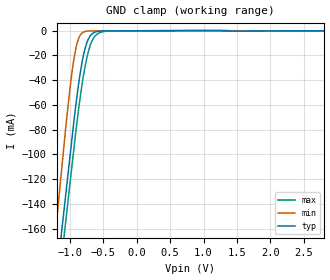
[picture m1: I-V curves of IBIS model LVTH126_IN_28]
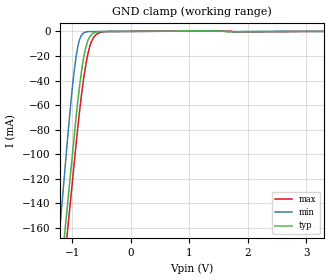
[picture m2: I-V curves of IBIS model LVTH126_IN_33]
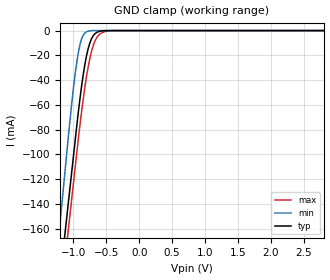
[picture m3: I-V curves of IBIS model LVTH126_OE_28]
| TEXAS INSTRUMENTS INCORPORATED
| Standard Linear and Logic Group
| IBIS Model of SN74LVTH126
| 3.3-V ABT QUADRUPLE BUS BUFFERS WITH 3-STATE OUTPUTS
| This file contains package information for the following:
|  TSSOP 14-pin (PW) package as [Component] LVTH126_PW
|  SOP 14-pin (NS) package as [Component] LVTH126_NS
|  TVSOP 14-pin (DGV) package as [Component] LVTH126_DGV
|  SSOP 14-pin (DB) package as [Component] LVTH126_DB
|  SOIC 14-pin (D) package as [Component] LVTH126_D
| This device can be powered at the following Vccs:
|  2.8 volt Vcc
|  3.3 volt Vcc
| This file provides unique models under the [Model Selector] for each Vcc.
| For operation at a specific Vcc, select the appropriate model after each
| [Model Selector] keyword.
[IBIS Ver]   3.2
[Comment char]  |_char
[File Name]   sn74lvth126.ibs
[File Rev]   1.1 | b_die
[Date]   June 13, 2002
[Source]   Data created from TI-SPICE simulations at TI-SLL.
[Notes]   The following is an IBIS list for the SN74LVTH126.
   Please contact sllibis@ti.com with questions and
   comments concerning SLL IBIS models.
   - Due to the fact that the device is 5-V input/output
   tolerant, the output model has some non-monotonic
   warnings.
   - C_comp values are taken at a different test condition
   than the Ci in data sheet.
   - Power clamp data has been deleted since there is no
   power clamp diode in the device.
   - Due to presence of BUS HOLD at input, GND-CLAMP curves
   have non-monotonic warnings.
[Disclaimer] Property of Texas Instruments Incorporated.  Unauthorized
   reproduction and/or distribution is strictly prohibited.
   This product is protected under copyright law.
   Created 2002, (C) Copyright 2002, Texas Instruments
   Incorporated, All Rights Reserved
   UNLESS THERE IS A SIGNED, WRITTEN AGREEMENT TO THE
   CONTRARY, TEXAS INSTRUMENTS (TI) IS PROVIDING THE IBIS
   MODELS  AND WITHOUT ANY WARRANTY, EXPRESSED OR
   IMPLIED. TI assumes no liability for:
   1) the accuracy of the IBIS models provided to your
   company;
   2) the proper functioning of these IBIS Models in your
   design or for any resulting applications; or
   3) infringement of patents, copyrights or intellectual
   property rights resulting from your use of these IBIS
   models.
   TI provides IBIS Models as a service to our customers.
   You and your company shall not distribute, sell or give
   these models to anyone else without prior written
   permission from TI.
   TI reserves the right to make changes to our products or
   to discontinue any semiconductor product or service
   without notice, and advises our customers to obtain the
   latest version of relevant information to verify, before
   placing orders, that the information being relied on is
   current.
   Please be aware that your receipt and use of the IBIS
   information provided shall serve as acceptance of these
   terms and conditions. If you do not accept these terms,
   you should return or destroy the IBIS models and any
   other accompanying information immediately.
| Component LVTH126_PW 14-pin TSSOP
[Component]   LVTH126_PW
[Manufacturer]  Texas Instruments, Inc.
[Package]
|   typ   min   max
R_pkg   3.200e-02   2.900e-02   3.500e-02
L_pkg   2.378e-09   2.170e-09   2.680e-09
C_pkg   3.140e-13   2.700e-13   3.350e-13
[Pin]   signal_name   model_name   R_pin   L_pin   C_pin
1   1OE   LVTH126_OE   3.300e-02   2.618e-09   3.300e-13
2   1A   LVTH126_IN   3.100e-02   2.313e-09   3.170e-13
3   1Y   LVTH126_OUT   3.000e-02   2.310e-09   3.140e-13
4   2OE   LVTH126_OE   3.100e-02   2.173e-09   2.720e-13
5   2A   LVTH126_IN   3.000e-02   2.204e-09   3.090e-13
6   2Y   LVTH126_OUT   3.200e-02   2.315e-09   3.170e-13
7   GND   GND   3.500e-02   2.680e-09   3.350e-13
8   3Y   LVTH126_OUT   3.300e-02   2.640e-09   3.330e-13
9   3A   LVTH126_IN   3.400e-02   2.347e-09   3.190e-13
10   3OE   LVTH126_OE   2.900e-02   2.277e-09   3.130e-13
11   4Y   LVTH126_OUT   3.100e-02   2.170e-09   2.700e-13
12   4A   LVTH126_IN   3.100e-02   2.244e-09   3.110e-13
13   4OE   LVTH126_OE   3.300e-02   2.343e-09   3.210e-13
14   VCC   POWER   3.500e-02   2.657e-09   3.320e-13
| Component LVTH126_NS 14-pin SOP
[Component]   LVTH126_NS
[Manufacturer]  Texas Instruments, Inc.
[Package]
|   typ   min   max
R_pkg   4.500e-02   3.900e-02   5.400e-02
L_pkg   3.796e-09   2.561e-09   4.952e-09
C_pkg   5.280e-13   2.880e-13   7.100e-13
[Pin]   signal_name   model_name   R_pin   L_pin   C_pin
1   1OE   LVTH126_OE   4.700e-02   4.867e-09   7.060e-13
2   1A   LVTH126_IN   5.100e-02   4.083e-09   5.920e-13
3   1Y   LVTH126_OUT   4.100e-02   2.915e-09   3.760e-13
4   2OE   LVTH126_OE   3.900e-02   2.561e-09   2.880e-13
5   2A   LVTH126_IN   4.100e-02   3.101e-09   4.300e-13
6   2Y   LVTH126_OUT   4.700e-02   4.047e-09   5.890e-13
7   GND   GND   5.100e-02   4.909e-09   7.000e-13
8   3Y   LVTH126_OUT   4.500e-02   4.784e-09   6.940e-13
9   3A   LVTH126_IN   5.400e-02   4.176e-09   5.970e-13
10   3OE   LVTH126_OE   3.900e-02   3.287e-09   4.490e-13
11   4Y   LVTH126_OUT   3.900e-02   2.586e-09   2.940e-13
12   4A   LVTH126_IN   4.000e-02   2.802e-09   3.710e-13
13   4OE   LVTH126_OE   4.900e-02   4.080e-09   5.930e-13
14   VCC   POWER   5.200e-02   4.952e-09   7.100e-13
| Component LVTH126_DGV 14-pin TVSOP
[Component]   LVTH126_DGV
[Manufacturer]  Texas Instruments, Inc.
[Package]
|   typ   min   max
R_pkg   3.500e-02   2.000e-02   4.500e-02
L_pkg   2.499e-09   2.077e-09   2.966e-09
C_pkg   3.610e-13   3.050e-13   4.160e-13
[Pin]   signal_name   model_name   R_pin   L_pin   C_pin
1   1OE   LVTH126_OE   2.700e-02   2.717e-09   3.730e-13
2   1A   LVTH126_IN   3.700e-02   2.434e-09   3.980e-13
3   1Y   LVTH126_OUT   3.400e-02   2.200e-09   3.160e-13
4   2OE   LVTH126_OE   2.000e-02   2.077e-09   3.090e-13
5   2A   LVTH126_IN   3.000e-02   2.147e-09   3.050e-13
6   2Y   LVTH126_OUT   4.200e-02   2.580e-09   4.080e-13
7   GND   GND   3.900e-02   2.921e-09   3.850e-13
8   3Y   LVTH126_OUT   3.300e-02   2.841e-09   3.800e-13
9   3A   LVTH126_IN   4.200e-02   2.611e-09   4.100e-13
10   3OE   LVTH126_OE   3.800e-02   2.331e-09   3.290e-13
11   4Y   LVTH126_OUT   2.600e-02   2.223e-09   3.190e-13
12   4A   LVTH126_IN   3.400e-02   2.259e-09   3.130e-13
13   4OE   LVTH126_OE   4.500e-02   2.681e-09   4.160e-13
14   VCC   POWER   4.200e-02   2.966e-09   3.860e-13
| Component LVTH126_DB 14-pin SSOP
[Component]   LVTH126_DB
[Manufacturer]  Texas Instruments, Inc.
[Package]
|   typ   min   max
R_pkg   4.400e-02   4.100e-02   4.600e-02
L_pkg   3.551e-09   3.258e-09   3.927e-09
C_pkg   4.020e-13   3.600e-13   4.210e-13
[Pin]   signal_name   model_name   R_pin   L_pin   C_pin
1   1OE   LVTH126_OE   4.600e-02   3.927e-09   4.080e-13
2   1A   LVTH126_IN   4.400e-02   3.587e-09   4.210e-13
3   1Y   LVTH126_OUT   4.100e-02   3.289e-09   3.980e-13
4   2OE   LVTH126_OE   4.200e-02   3.258e-09   3.600e-13
5   2A   LVTH126_IN   4.100e-02   3.286e-09   4.030e-13
6   2Y   LVTH126_OUT   4.400e-02   3.586e-09   4.210e-13
7   GND   GND   4.600e-02   3.927e-09   4.080e-13
8   3Y   LVTH126_OUT   4.600e-02   3.927e-09   4.080e-13
9   3A   LVTH126_IN   4.400e-02   3.586e-09   4.210e-13
10   3OE   LVTH126_OE   4.100e-02   3.286e-09   4.030e-13
11   4Y   LVTH126_OUT   4.300e-02   3.258e-09   3.600e-13
12   4A   LVTH126_IN   4.100e-02   3.289e-09   3.980e-13
13   4OE   LVTH126_OE   4.400e-02   3.587e-09   4.210e-13
14   VCC   POWER   4.600e-02   3.927e-09   4.080e-13
| Component LVTH126_D 14-pin SOIC
[Component]   LVTH126_D
[Manufacturer]  Texas Instruments, Inc.
[Package]
|   typ   min   max
R_pkg   3.100e-02   2.800e-02   3.400e-02
L_pkg   3.109e-09   2.462e-09   3.889e-09
C_pkg   4.730e-13   3.630e-13   6.280e-13
[Pin]   signal_name   model_name   R_pin   L_pin   C_pin
1   1OE   LVTH126_OE   3.300e-02   3.854e-09   6.220e-13
2   1A   LVTH126_IN   3.200e-02   3.188e-09   4.730e-13
3   1Y   LVTH126_OUT   2.800e-02   2.462e-09   3.770e-13
4   2OE   LVTH126_OE   3.100e-02   2.596e-09   3.630e-13
5   2A   LVTH126_IN   2.800e-02   2.521e-09   3.720e-13
6   2Y   LVTH126_OUT   3.400e-02   3.250e-09   4.760e-13
7   GND   GND   3.400e-02   3.889e-09   6.280e-13
8   3Y   LVTH126_OUT   3.400e-02   3.889e-09   6.280e-13
9   3A   LVTH126_IN   3.400e-02   3.250e-09   4.760e-13
10   3OE   LVTH126_OE   2.800e-02   2.521e-09   3.720e-13
11   4Y   LVTH126_OUT   3.100e-02   2.596e-09   3.640e-13
12   4A   LVTH126_IN   2.800e-02   2.462e-09   3.770e-13
13   4OE   LVTH126_OE   3.200e-02   3.188e-09   4.730e-13
14   VCC   POWER   3.300e-02   3.854e-09   6.220e-13
| Model LVTH126_IN
[Model Selector]   LVTH126_IN
LVTH126_IN_28   2.8 volt Vcc
LVTH126_IN_33   3.3 volt Vcc
| Model LVTH126_OE
[Model Selector]   LVTH126_OE
LVTH126_OE_28   2.8 volt Vcc
LVTH126_OE_33   3.3 volt Vcc
| Model LVTH126_OUT
[Model Selector]   LVTH126_OUT
LVTH126_OUT_28   2.8 volt Vcc
LVTH126_OUT_33   3.3 volt Vcc
| Models and submodels in the file (6): LVTH126_IN_28 (Input), LVTH126_IN_33 (Input), LVTH126_OE_28 (Input), LVTH126_OE_33 (Input), LVTH126_OUT_28 (3-state), LVTH126_OUT_33 (3-state)
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[Model]   LVTH126_IN_28
Model_type  Input
Vinl=0.8
Vinh=2.0
| variable   typ   min   max
C_comp   1.60pF   1.29pF   1.95pF
[Temperature Range]   40   -40   100
| Ambient temperature   25   -40   85
[Voltage range]   2.8   2.7   2.9
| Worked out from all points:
|   GND clamp passes 1 mA (typ) near -0.62 V on its own axis
[GND Clamp]
| LVTH126_IN_28
|   Voltage   I(typ)   I(min)   I(max)
-5.5V     -2.408A    -2.647A    -2.409A
-1.22V    -209.4mA   -166.1mA   -230.4mA
-1.205V   -202.1mA   -157.7mA   -223.2mA
-1.125V   -163.2mA   -113.1mA   -184.6mA
-1.075V   -138.9mA   -85.4mA    -160.5mA
-975mV    -90.32mA   -36.3mA    -112.3mA
-900mV    -55.42mA   -11.62mA   -76.73mA
-800mV    -20.4mA    -1.144mA   -37.12mA
-675mV    -2.832mA   -139.6uA   -8.888mA
-575mV    -458.4uA   -111.4uA   -2.116mA
-425mV    -91.65uA   -80.03uA   -193.6uA
2.8V      16.5pA     10.34pA    -1.624nA
[Model]   LVTH126_IN_33
Model_type  Input
Vinl=0.8
Vinh=2.34
| variable   typ   min   max
C_comp   1.60pF   1.28pF   1.93pF
[Temperature Range]   40   -40   100
| Ambient temperature   25   -40   85
[Voltage range]   3.3   3   3.6
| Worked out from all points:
|   GND clamp passes 1 mA (typ) near -0.62 V on its own axis
[GND Clamp]
| LVTH126_IN_33
|   Voltage   I(typ)   I(min)   I(max)
-5.5V     -2.408A    -2.647A    -2.409A
-1.22V    -209.4mA   -166.1mA   -230.4mA
-1.125V   -163.2mA   -113.2mA   -184.6mA
-1.075V   -138.9mA   -85.42mA   -160.5mA
-975mV    -90.33mA   -36.31mA   -112.3mA
-900mV    -55.43mA   -11.64mA   -76.74mA
-825mV    -27.57mA   -2.158mA   -45.91mA
-775mV    -14.79mA   -631.5uA   -29.62mA
-725mV    -6.832mA   -223.9uA   -17.14mA
-650mV    -1.834mA   -140.7uA   -6.297mA
-405mV    -96.3uA    -83.61uA   -155.7uA
3.3V      19.45pA    12.56pA    -1.138uA
[Model]   LVTH126_OE_28
Model_type  Input
Vinl=0.8
Vinh=2.0
| variable   typ   min   max
C_comp   1.60pF   1.34pF   1.99pF
[Temperature Range]   40   -40   100
| Ambient temperature   25   -40   85
[Voltage range]   2.8   2.7   2.9
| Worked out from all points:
|   GND clamp passes 1 mA (typ) near -0.62 V on its own axis
[GND Clamp]
| LVTH126_OE_28
|   Voltage   I(typ)   I(min)   I(max)
-5.5V     -2.407A    -2.647A    -2.408A
-1.22V    -209.3mA   -166mA     -230.3mA
-1.205V   -202mA     -157.5mA   -223mA
-1.125V   -163.1mA   -113mA     -184.4mA
-1.075V   -138.8mA   -85.24mA   -160.3mA
-975mV    -90.17mA   -36.12mA   -112.1mA
-900mV    -55.28mA   -11.44mA   -76.59mA
-800mV    -20.27mA   -984.6uA   -37mA
-675mV    -2.699mA   -6.758uA   -8.774mA
-575mV    -336.8uA   -57.38nA   -2.013mA
-425mV    -3.297uA   -110.8pA   -103uA
2.8V      13.7pA     7.338pA    757.3pA
